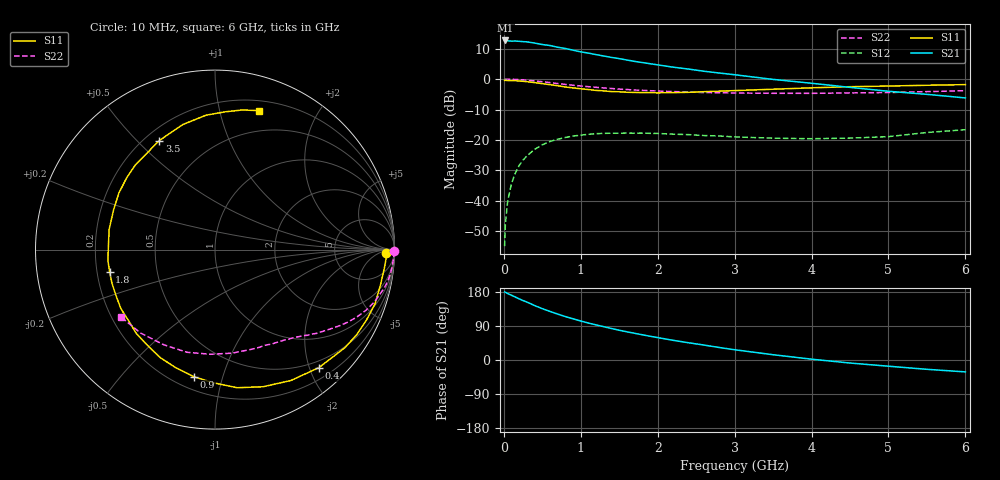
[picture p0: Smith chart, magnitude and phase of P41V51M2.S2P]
! SIEMENS Small Signal Semiconductors
! BFP182
! Si NPN RF Bipolar Junction Transistor in SOT143
! VCE = 1.5 V  IC = 1.2 mA
! Common Emitter S-Parameters:  March  1996
# GHz  S  MA  R  50
!  f  S11  S21  S12  S22
! GHz  MAG  ANG  MAG  ANG  MAG  ANG  MAG  ANG
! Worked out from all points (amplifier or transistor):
!   36 points, 10 MHz to 6 GHz, reference 50 ohm
!   highest |S21| = 12.7 dB at 20 MHz (marker M1)
!   |S21| within 3 dB of that: start of sweep to 864.3 MHz
!   unconditionally stable (mu >= 1): 2.487 GHz to end of sweep
!   at 250 MHz: K = 0.10, MSG = 19.5 dB, |S12| = -26.6 dB
!   at 1.4 GHz: K = 0.57, MSG = 12.4 dB, |S12| = -17.8 dB
!   at 6 GHz: K = 1.09, MAG = 3.4 dB, |S12| = -16.6 dB
!   S11 on the Smith chart (normalised r, x): 10 MHz: 37, -15; 400 MHz: 0.38, -2.15; 900 MHz: 0.28, -0.81; 1.8 GHz: 0.25, -0.10; 3.5 GHz: 0.26, +0.58; 6 GHz: 0.29, +1.32
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0.01  0.9543 -1.1  4.23 179.5  0.0018 92.2  0.9973 -0.5
0.02  0.9559 -2.5  4.317 178.8  0.0042 86.0  0.9968 -1.0
0.05  0.9491 -6.3  4.269 175.5  0.0099 85.2  0.9968 -2.4
0.1  0.9426 -12.3  4.204 170.8  0.0193 81.9  0.9923 -4.8
0.15  0.9416 -18.7  4.225 166.0  0.0287 78.2  0.9879 -7.3
0.25  0.9208 -31.0  4.126 156.8  0.0467 71.3  0.9715 -11.9
0.3  0.9068 -37.1  4.097 152.8  0.0548 67.8  0.9585 -14.1
0.4  0.876 -48.7  3.91 143.7  0.0701 60.5  0.934 -18.3
0.5  0.8429 -59.9  3.703 135.5  0.0833 54.2  0.9056 -22.0
0.6  0.8099 -70.6  3.562 128.2  0.0945 48.4  0.876 -25.3
0.8  0.7422 -90.6  3.185 114.5  0.1099 38.1  0.8181 -31.0
0.9  0.718 -99.4  2.987 108.7  0.1159 34.0  0.7928 -33.3
1.1  0.6741 -117.1  2.671 97.4  0.1241 26.4  0.7507 -37.5
1.3  0.6407 -133.2  2.395 87.8  0.1284 19.9  0.7164 -41.1
1.5  0.6191 -147.8  2.171 78.5  0.1291 15.0  0.6854 -44.4
1.8  0.6 -168.1  1.873 66.5  0.1296 9.4  0.6543 -48.8
2.2  0.6005 169.2  1.571 52.0  0.1246 3.6  0.624 -55.4
2.8  0.6338 141.1  1.26 33.0  0.1163 -1.0  0.5974 -65.9
3.5  0.6822 117.1  0.989 13.9  0.1071 -0.2  0.5849 -80.5
4.5  0.7505 93.8  0.732 -8.0  0.1074 6.9  0.5931 -105.4
5.5  0.7928 78.9  0.562 -24.6  0.1327 13.7  0.623 -131.8
6  0.8118 72.5  0.491 -31.4  0.1476 12.1  0.6451 -144.6
